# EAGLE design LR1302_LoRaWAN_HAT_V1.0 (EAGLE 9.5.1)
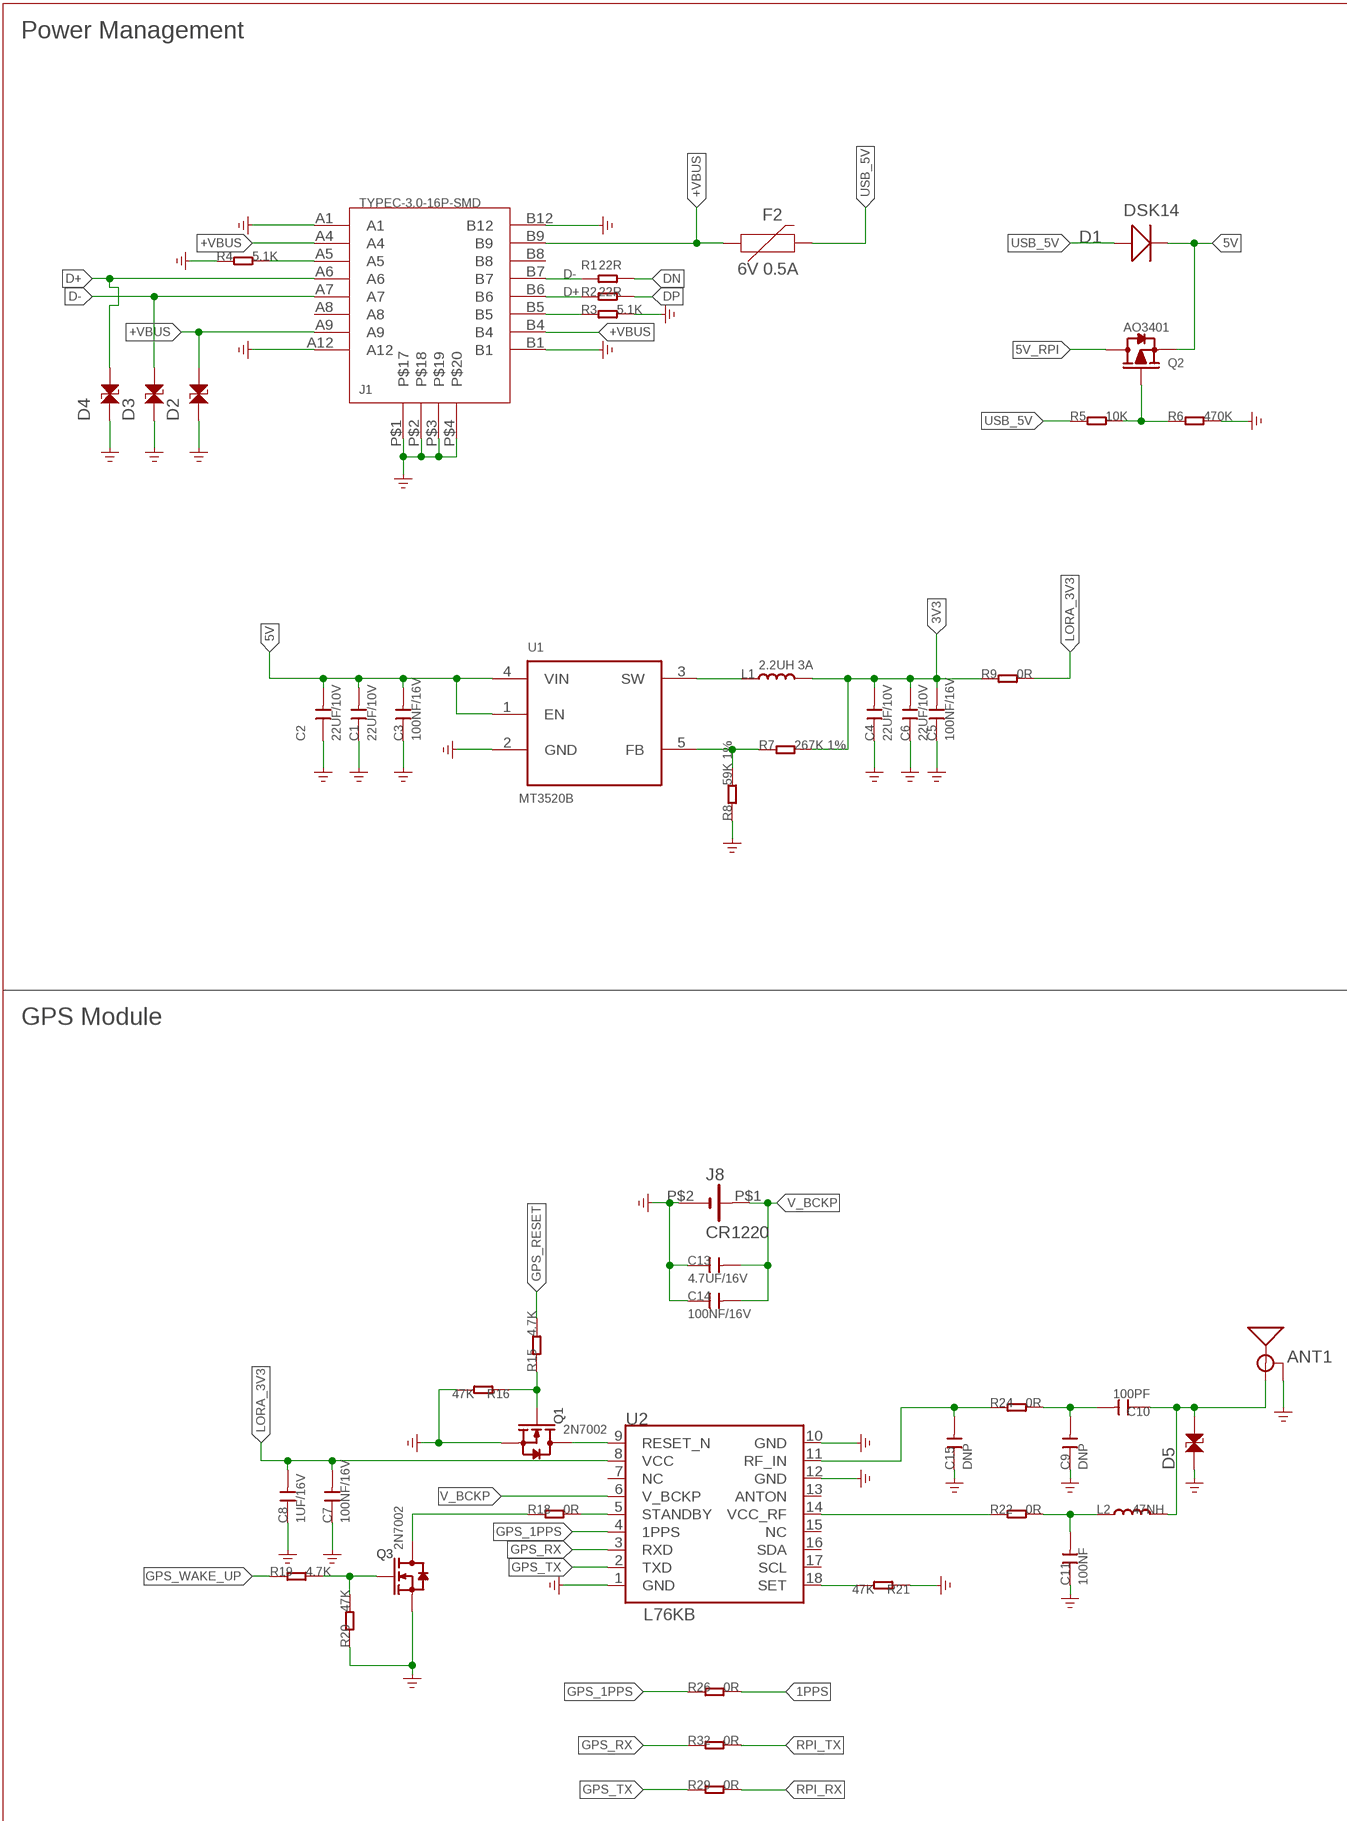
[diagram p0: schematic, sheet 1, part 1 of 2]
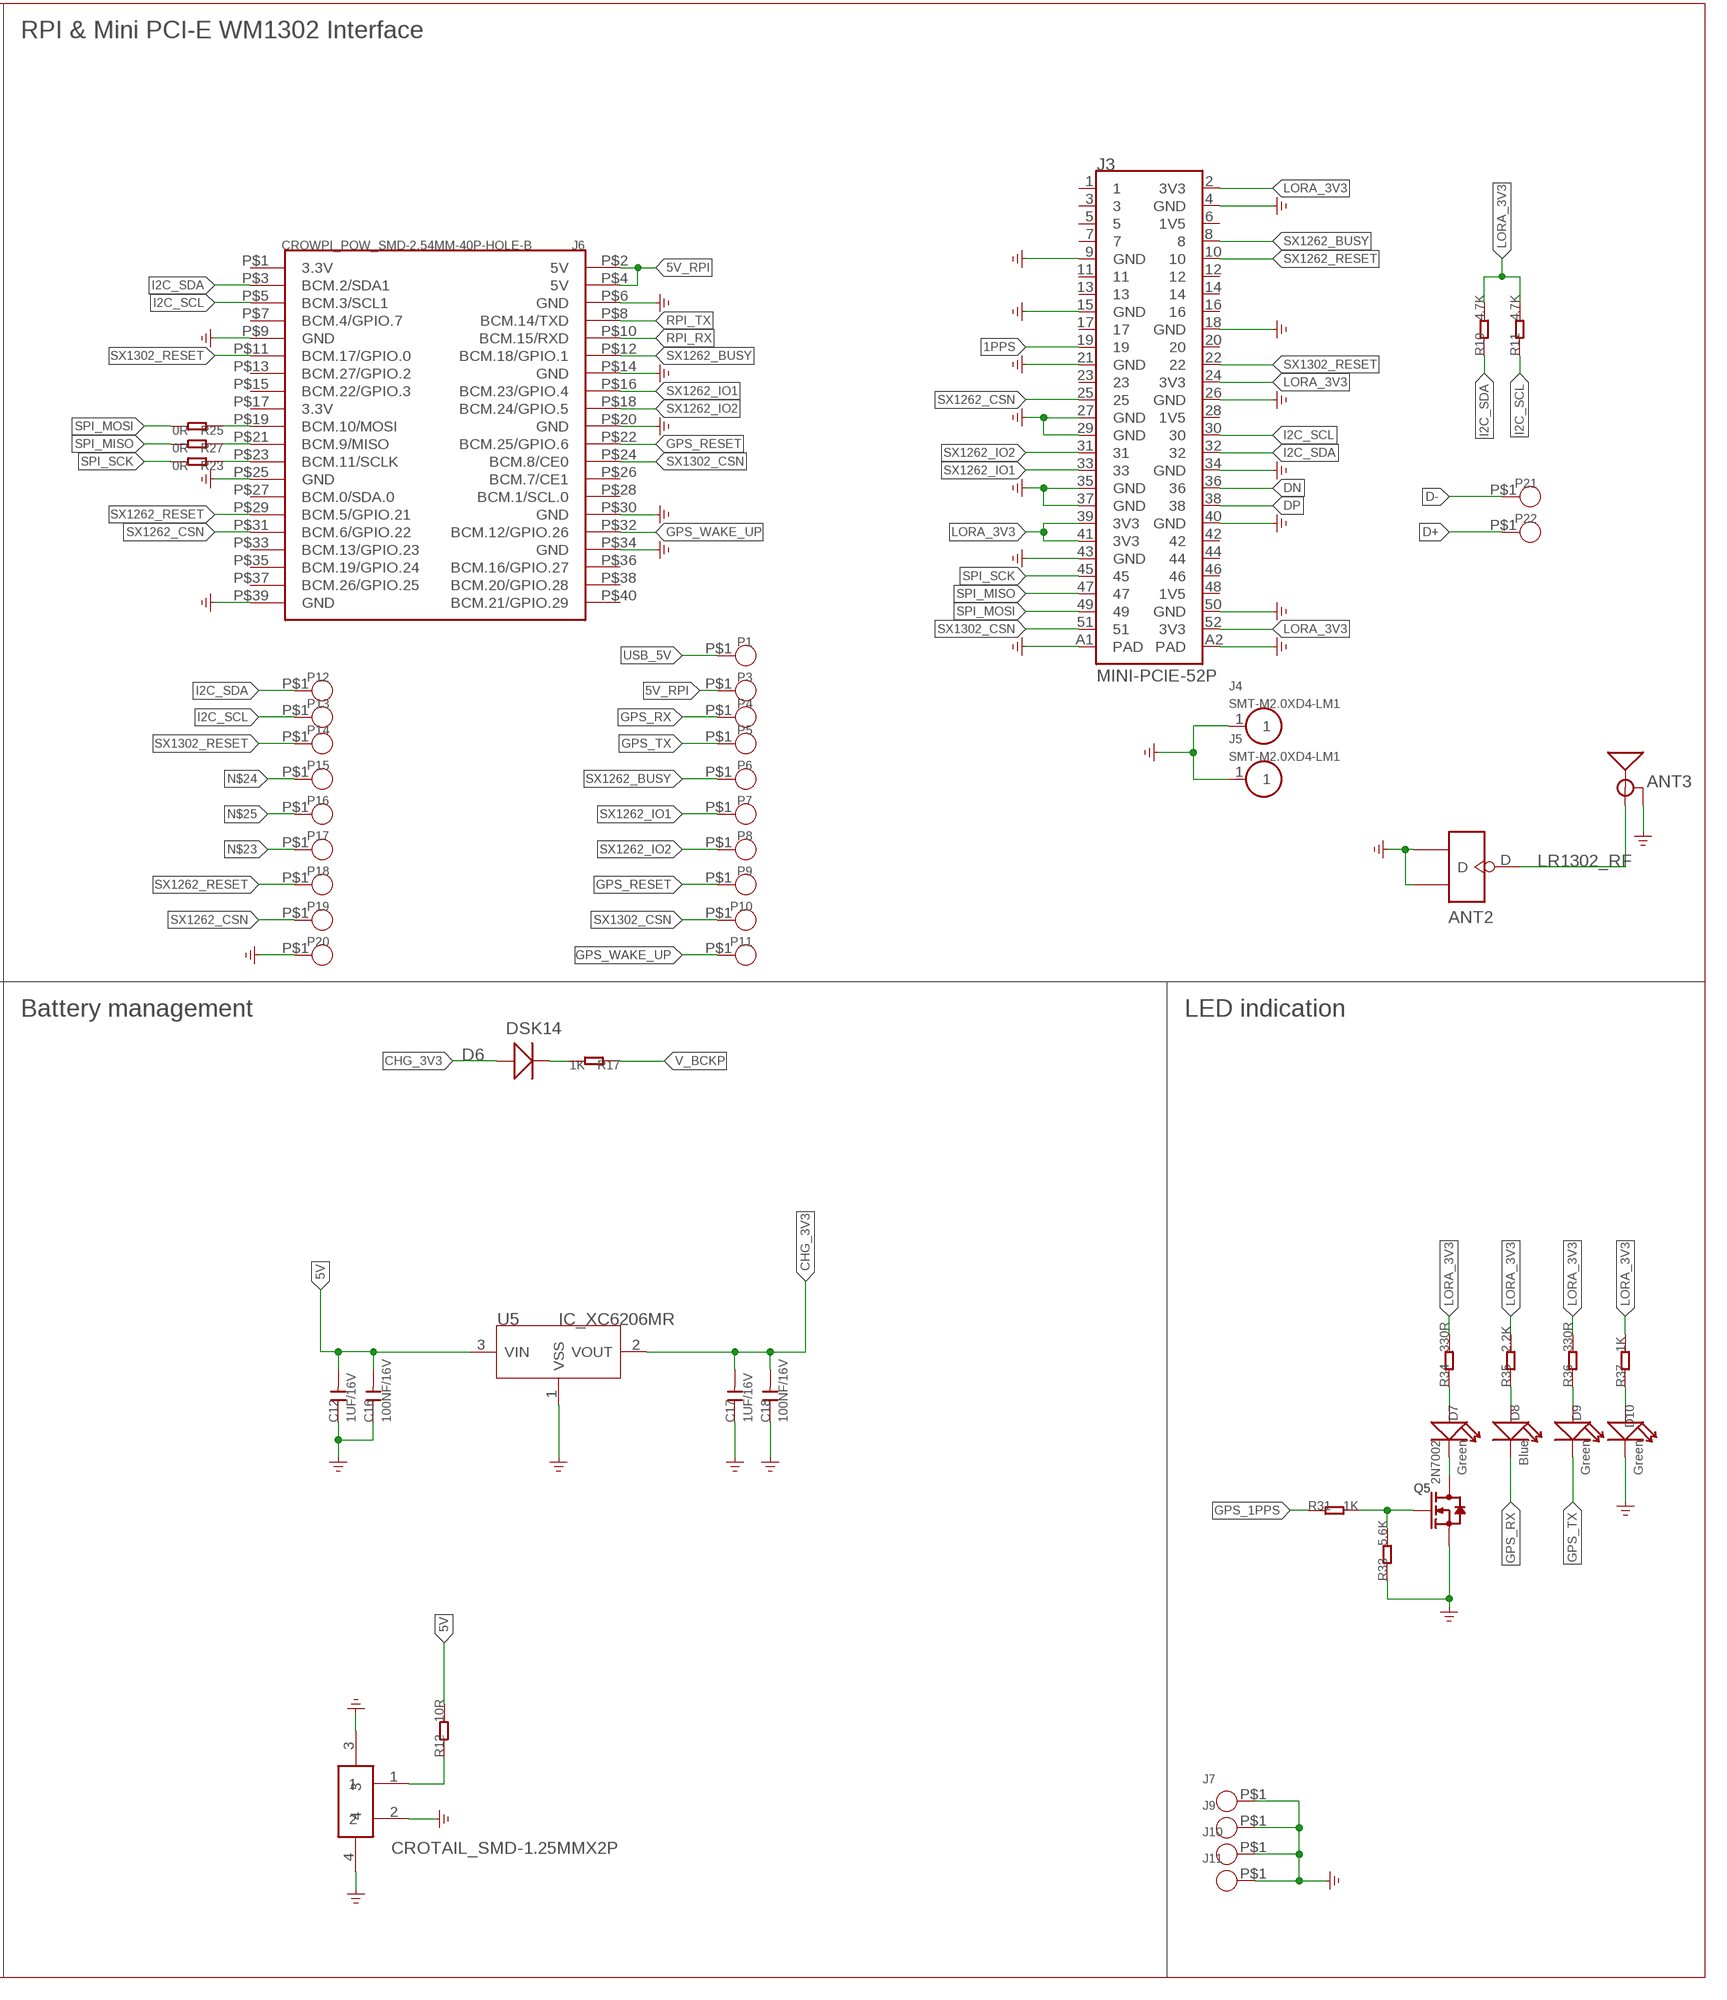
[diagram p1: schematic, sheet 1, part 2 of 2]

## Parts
ANT1  ANTENNA-SMA-GROUNDEDEDGE_SMA  [SMA-EDGE]
ANT2  CONNECTOR-NEW_ANTENNA-U-FL  [CONNECTOR-NEW_U-FL3P-SMD-2.6X2.6X1.0MM]
ANT3  ANTENNA-SMA-GROUNDEDEDGE_SMA  [SMA-EDGE]
C1  22UF/10V  C0805  [C0805]
C2  22UF/10V  C0805  [C0805]
C3  100NF/16V  C0603  [C0603]
C4  22UF/10V  C0805  [C0805]
C5  100NF/16V  C0603  [C0603]
C6  22UF/10V  C0805  [C0805]
C7  100NF/16V  C0603  [C0603]
C8  1UF/16V  C0603  [C0603]
C9  DNP  C0603  [C0603]
C10  100PF  C0603  [C0603]
C11  100NF  C0603  [C0603]
C12  1UF/16V  C0603  [C0603]
C13  4.7UF/16V  C0603  [C0603]
C14  100NF/16V  C0603  [C0603]
C15  DNP  C0603  [C0603]
C16  100NF/16V  C0603  [C0603]
C17  1UF/16V  C0603  [C0603]
C18  100NF/16V  C0603  [C0603]
D1  DSK14  DIODE  [D_SOD123FL]
D2  LXES15AAA1-153  [0402-ESD]
D3  LXES15AAA1-153  [0402-ESD]
D4  LXES15AAA1-153  [0402-ESD]
D5  LXES15AAA1-153  [0402-ESD]
D6  DSK14  DIODE  [D_SOD123FL]
D7  Green  LED-SMT0603  [LED0603]
D8  Blue  LED-SMT0603  [LED0603]
D9  Green  LED-SMT0603  [LED0603]
D10  Green  LED-SMT0603  [LED0603]
F2  6V 0.5A  PPTC_6V500MA  [0805]
J1  TYPEC-3.0-16P-SMD  [KEVIN_3.0TYPEC-SMD]
J2  CROTAIL_SMD-1.25MMX2P  [CROTAIL_SMD-1.25MMX2P]
J3  MINI-PCIE-52P  [MPCI-E0.8MM-52P-SMD]
J4  SMT-M2.0XD4-LM1  [SMD-M2.0XD4.0-LM]
J5  SMT-M2.0XD4-LM1  [SMD-M2.0XD4.0-LM]
J6  CROWPI_POW_SMD-2.54MM-40P-HOLE-B  [CROWPI_POW_SMD-2.54MM-40P-HOLE-B]
J7  PAD-HOLE  [PAD-THOD600X280]
J8  CR1220  CR1220LFCR1220-SMD  [CR1220-SMD]
J9  PAD-HOLE  [PAD-THOD600X280]
J10  PAD-HOLE  [PAD-THOD600X280]
J11  PAD-HOLE  [PAD-THOD600X280]
L1  2.2UH 3A  LL0420  [L0420]
L2  47NH  L0603  [L0603]
P1  TEST_PADPAD-1.5MM  [TEST_PAD-1.5MM]
P3  TEST_PADPAD-1.5MM  [TEST_PAD-1.5MM]
P4  TEST_PADPAD-1.5MM  [TEST_PAD-1.5MM]
P5  TEST_PADPAD-1.5MM  [TEST_PAD-1.5MM]
P6  TEST_PADPAD-1.5MM  [TEST_PAD-1.5MM]
P7  TEST_PADPAD-1.5MM  [TEST_PAD-1.5MM]
P8  TEST_PADPAD-1.5MM  [TEST_PAD-1.5MM]
P9  TEST_PADPAD-1.5MM  [TEST_PAD-1.5MM]
P10  TEST_PADPAD-1.5MM  [TEST_PAD-1.5MM]
P11  TEST_PADPAD-1.5MM  [TEST_PAD-1.5MM]
P12  TEST_PADPAD-1.5MM  [TEST_PAD-1.5MM]
P13  TEST_PADPAD-1.5MM  [TEST_PAD-1.5MM]
P14  TEST_PADPAD-1.5MM  [TEST_PAD-1.5MM]
P15  TEST_PADPAD-1.5MM  [TEST_PAD-1.5MM]
P16  TEST_PADPAD-1.5MM  [TEST_PAD-1.5MM]
P17  TEST_PADPAD-1.5MM  [TEST_PAD-1.5MM]
P18  TEST_PADPAD-1.5MM  [TEST_PAD-1.5MM]
P19  TEST_PADPAD-1.5MM  [TEST_PAD-1.5MM]
P20  TEST_PADPAD-1.5MM  [TEST_PAD-1.5MM]
P21  TEST_PADPAD-1.5MM  [TEST_PAD-1.5MM]
P22  TEST_PADPAD-1.5MM  [TEST_PAD-1.5MM]
Q1  2N7002  MOSFET-NSOT23  [MOS_SOT23]
Q2  AO3401  MOSFET-PSOT23  [PMOS_SOT23]
Q3  2N7002  MOSFET-NSOT23  [MOS_SOT23]
Q5  2N7002  MOSFET-NSOT23  [MOS_SOT23]
R1  22R  R0603  [R0603]
R2  22R  R0603  [R0603]
R3  5.1K  R0603  [R0603]
R4  5.1K  R0603  [R0603]
R5  10K  R0603  [R0603]
R6  470K  R0603  [R0603]
R7  267K 1%  R0603  [R0603]
R8  59K 1%  R0603  [R0603]
R9  0R  R0603  [R0603]
R10  4.7K  R0603  [R0603]
R11  4.7K  R0603  [R0603]
R12  10R  R0603  [R0603]
R15  4.7K  R0603  [R0603]
R16  47K  R0603  [R0603]
R17  1K  R0603  [R0603]
R18  0R  R0603  [R0603]
R19  4.7K  R0603  [R0603]
R20  47K  R0603  [R0603]
R21  47K  R0603  [R0603]
R22  0R  R0603  [R0603]
R23  0R  R0603  [R0603]
R24  0R  R0603  [R0603]
R25  0R  R0603  [R0603]
R26  0R  R0603  [R0603]
R27  0R  R0603  [R0603]
R29  0R  R0603  [R0603]
R31  1K  R0603  [R0603]
R32  0R  R0603  [R0603]
R33  5.6K  R0603  [R0603]
R34  330R  R0603  [R0603]
R35  2.2K  R0603  [R0603]
R36  330R  R0603  [R0603]
R37  1K  R0603  [R0603]
U1  MT3520B  [IC_SOT23-5]
U2  L76KB  [LCC-18]
U5  IC_XC6206MR  [IC_SOT23]

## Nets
1PPS: J3.19 R26.2
3V3: C4.2 C5.2 C6.2 L1.2 R7.2 R9.1
5V: C1.2 C2.2 C3.2 C12.2 C16.2 D1.- Q2.2(S) R12.2 U1.1(EN) U1.4(VIN) U5.3(VIN)
5V_RPI: J6.P$2(5V) J6.P$4(5V) P3.P$1 Q2.3(D)
+VBUS: D2.2 F2.1 J1.A4 J1.A9 J1.B4 J1.B9
CHG_3V3: C17.2 C18.2 D6.+ U5.2(VOUT)
D+: D4.2 J1.A6 J1.B6 P22.P$1 R2.1
D-: D3.2 J1.A7 J1.B7 P21.P$1 R1.1
DN: J3.36 R1.2
DP: J3.38 R2.2
GND: ANT1.GND@0(GND) ANT1.GND@1(GND) ANT1.GND@2(GND) ANT1.GND@3(GND) ANT2.GND1 ANT2.GND2 ANT3.GND@0(GND) ANT3.GND@1(GND) ANT3.GND@2(GND) ANT3.GND@3(GND) C1.1 C2.1 C3.1 C4.1 C5.1 C6.1 C7.1 C8.1 C9.1 C11.1 C12.1 C13.1 C14.1 C15.1 C16.1 C17.1 C18.1 D2.1 D3.1 D4.1 D5.1 D10.- J1.A1 J1.A12 J1.B1 J1.B12 J1.P$1 J1.P$2 J1.P$3 J1.P$4 J2.2 J2.3 J2.4 J3.4(GND) J3.9(GND) J3.15(GND) J3.18(GND) J3.21(GND) J3.26(GND) J3.27(GND) J3.29(GND) J3.34(GND) J3.35(GND) J3.37(GND) J3.40(GND) J3.43(GND) J3.50(GND) J3.A1(PAD) J3.A2(PAD) J4.1 J5.1 J6.P$6(GND) J6.P$9(GND) J6.P$14(GND) J6.P$20(GND) J6.P$25(GND) J6.P$30(GND) J6.P$34(GND) J6.P$39(GND) J7.P$1 J8.P$2(-) J9.P$1 J10.P$1 J11.P$1 P20.P$1 Q1.2(S) Q3.2(S) Q5.2(S) R3.2 R4.1 R6.2 R8.1 R16.2 R20.1 R21.1 R33.1 U1.2(GND) U2.1(GND) U2.10(GND) U2.12(GND) U5.1(VSS)
GPS_1PPS: R26.1 R31.1 U2.4(1PPS)
GPS_RESET: J6.P$22(BCM.25/GPIO.6) P9.P$1 R15.2
GPS_RX: D8.- P4.P$1 R32.1 U2.3(RXD)
GPS_TX: D9.- P5.P$1 R29.1 U2.2(TXD)
GPS_WAKE_UP: J6.P$32(BCM.12/GPIO.26) P11.P$1 R19.1
I2C_SCL: J3.30 J6.P$5(BCM.3/SCL1) P13.P$1 R11.1
I2C_SDA: J3.32 J6.P$3(BCM.2/SDA1) P12.P$1 R10.1
LORA_3V3: C7.2 C8.2 J3.2(3V3) J3.24(3V3) J3.39(3V3) J3.41(3V3) J3.52(3V3) R9.2 R10.2 R11.2 R34.2 R35.2 R36.2 R37.2 U2.8(VCC)
LR1302_RF: ANT2.D ANT3.SIG(SIGNAL)
N$1: J1.B5 R3.1
N$2: J1.A5 R4.2
N$3: L1.1 U1.3(SW)
N$4: R7.1 R8.2 U1.5(FB)
N$5: Q2.1(G) R5.2 R6.1
N$6: J2.1 R12.1
N$11: Q1.3(D) U2.9(RESET_N)
N$12: Q1.1(G) R15.1 R16.1
N$13: D6.- R17.2
N$14: R18.2 U2.5(STANDBY)
N$15: R21.2 U2.18(SET)
N$16: Q3.3(D) R18.1
N$17: Q3.1(G) R19.2 R20.2
N$18: C15.2 R24.1 U2.11(RF_IN)
N$19: C9.2 C10.2 R24.2
N$20: ANT1.SIG(SIGNAL) C10.1 D5.2 L2.2
N$21: R22.1 U2.14(VCC_RF)
N$22: C11.2 L2.1 R22.2
N$23: J6.P$23(BCM.11/SCLK) P17.P$1 R23.1
N$24: J6.P$19(BCM.10/MOSI) P15.P$1 R25.1
N$25: J6.P$21(BCM.9/MISO) P16.P$1 R27.1
N$27: Q5.1(G) R31.2 R33.2
N$28: D7.+ R34.1
N$29: D7.- Q5.3(D)
N$30: D8.+ R35.1
N$31: D10.+ R37.1
N$32: D9.+ R36.1
RPI_RX: J6.P$10(BCM.15/RXD) R29.2
RPI_TX: J6.P$8(BCM.14/TXD) R32.2
SPI_MISO: J3.47 R27.2
SPI_MOSI: J3.49 R25.2
SPI_SCK: J3.45 R23.2
SX1262_BUSY: J3.8 J6.P$12(BCM.18/GPIO.1) P6.P$1
SX1262_CSN: J3.25 J6.P$31(BCM.6/GPIO.22) P19.P$1
SX1262_IO1: J3.33 J6.P$16(BCM.23/GPIO.4) P7.P$1
SX1262_IO2: J3.31 J6.P$18(BCM.24/GPIO.5) P8.P$1
SX1262_RESET: J3.10 J6.P$29(BCM.5/GPIO.21) P18.P$1
SX1302_CSN: J3.51 J6.P$24(BCM.8/CE0) P10.P$1
SX1302_RESET: J3.22 J6.P$11(BCM.17/GPIO.0) P14.P$1
USB_5V: D1.+ F2.2 P1.P$1 R5.1
V_BCKP: C13.2 C14.2 J8.P$1(+) R17.1 U2.6(V_BCKP)
Unconnected: J1.A8 J1.B8 J3.1 J3.3 J3.5 J3.6(1V5) J3.7 J3.11 J3.12 J3.13 J3.14 J3.16 J3.17 J3.20 J3.23 J3.28(1V5) J3.42 J3.44 J3.46 J3.48(1V5) J6.P$1(3.3V) J6.P$7(BCM.4/GPIO.7) J6.P$13(BCM.27/GPIO.2) J6.P$15(BCM.22/GPIO.3) J6.P$17(3.3V) J6.P$26(BCM.7/CE1) J6.P$27(BCM.0/SDA.0) J6.P$28(BCM.1/SCL.0) J6.P$33(BCM.13/GPIO.23) J6.P$35(BCM.19/GPIO.24) J6.P$36(BCM.16/GPIO.27) J6.P$37(BCM.26/GPIO.25) J6.P$38(BCM.20/GPIO.28) J6.P$40(BCM.21/GPIO.29) U2.7(NC) U2.13(ANTON) U2.15(NC) U2.16(SDA) U2.17(SCL)

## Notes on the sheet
- Power Management | RPI & Mini PCI-E WM1302 Interface
- GPS Module | Battery management | LED indication

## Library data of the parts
ANT1 ANT3 = WM1302_Raspberry_Pi _Hat:ANTENNA-SMA-GROUNDED: SMA Antenna Connector w/ Ground; PROD_ID: CONN-08289
ANT2 = WM1302_Raspberry_Pi _Hat:CONNECTOR-NEW_ANTENNA-U-FL: 320110048
C1 C2 C4 C6 = WM1302_Raspberry_Pi _Hat:C0805
C3 C5 C7-C18 = WM1302_Raspberry_Pi _Hat:C0603
D1 D6 = WM1302_Raspberry_Pi _Hat:DIODE*
D2-D5 = WM1302_Raspberry_Pi _Hat:LXES15AAA1-153
D7-D10 = WM1302_Raspberry_Pi _Hat:LED-SMT*
F2 = WM1302_Raspberry_Pi _Hat:PPTC: Resettable Fuse PPTC; PROD_ID: RES-13945
J1 = WM1302_Raspberry_Pi _Hat:TYPEC-3.0-16P-SMD
J2 = WM1302_Raspberry_Pi _Hat:CROTAIL_SMD-1.25MMX2P
J3 = WM1302_Raspberry_Pi _Hat:MINI-PCIE-52P
J4 J5 = WM1302_Raspberry_Pi _Hat:SMT-M2.0XD4-LM1
J6 = WM1302_Raspberry_Pi _Hat:CROWPI_POW_SMD-2.54MM-40P-HOLE-B
J7 J9-J11 = WM1302_Raspberry_Pi _Hat:PAD-HOLE
J8 = WM1302_Raspberry_Pi _Hat:CR1220LF: Battery Holder, SMT, 12mm
L1 L2 = WM1302_Raspberry_Pi _Hat:L*
P1 P3-P22 = WM1302_Raspberry_Pi _Hat:TEST_PAD*
Q1 Q3 Q5 = WM1302_Raspberry_Pi _Hat:MOSFET-N*: IRLL014: http://www.vishay.com/docs/91319/sihll014.pdf
Q2 = WM1302_Raspberry_Pi _Hat:MOSFET-P: IRLL014: http://www.vishay.com/docs/91319/sihll014.pdf
R1-R12 R15-R27 R29 R31-R37 = WM1302_Raspberry_Pi _Hat:R0603
U1 = WM1302_Raspberry_Pi _Hat:MT3520B
U2 = WM1302_Raspberry_Pi _Hat:L76KB
U5 = WM1302_Raspberry_Pi _Hat:IC_XC6206: LOW ESR Cap.Compatible Positive Voltage Regulators

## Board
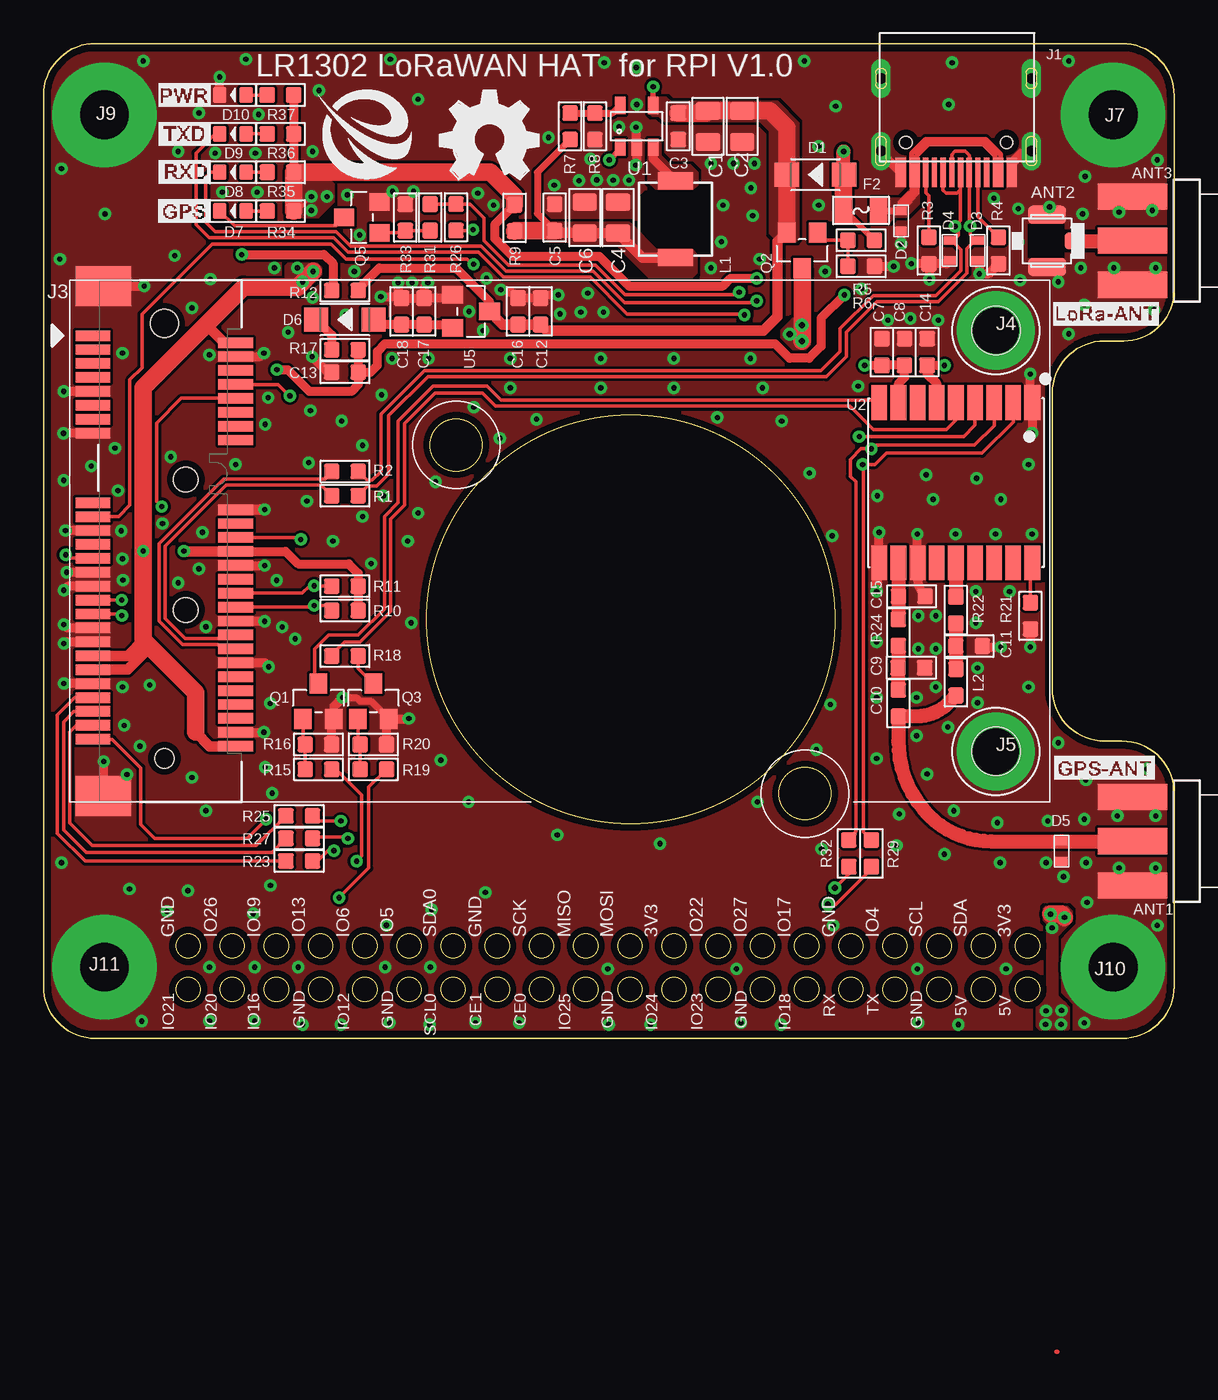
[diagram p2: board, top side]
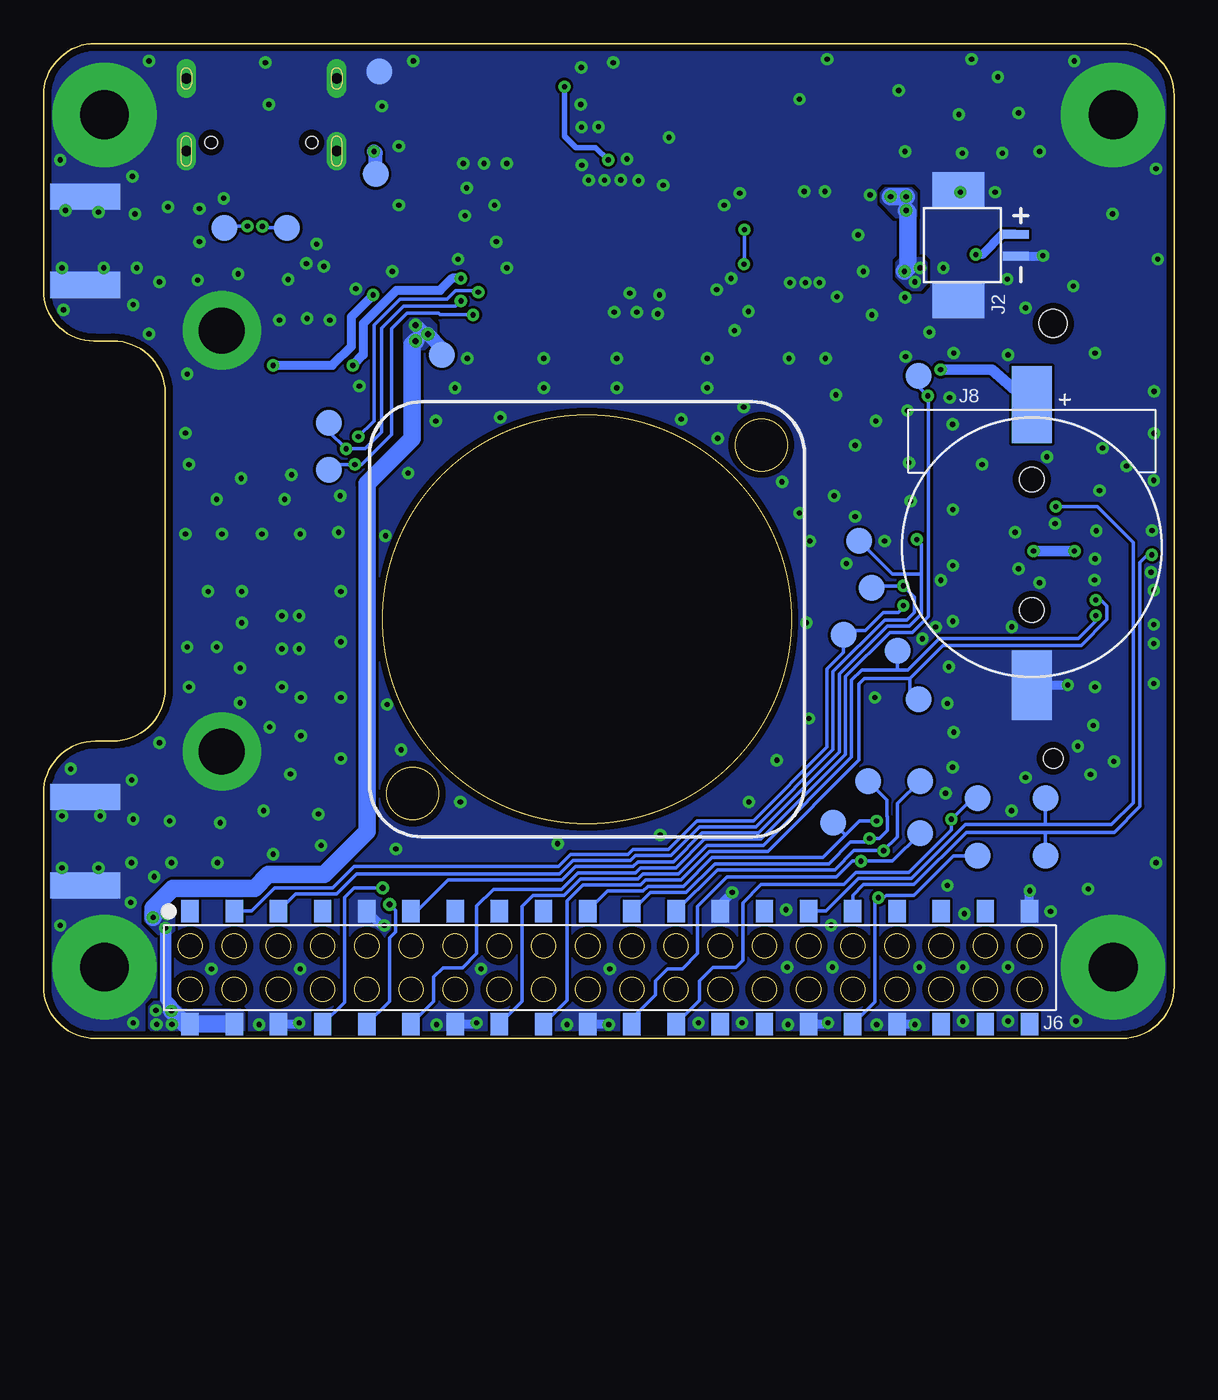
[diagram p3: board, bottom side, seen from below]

Size 65 x 57.2 mm. Coordinates in mm from the lower left corner, seen from the top.
Outline: 0,3 0,54.2 arc-90 3,57.2 62,57.2 arc-90 65,54.2 65,43 arc-90 62.1,40.1 61,40.1 arc90 58,37.1 58,20.1 arc90 61,17.1 62,17.1 arc-90 65,14.1 65,3 arc-90 62,0 3,0 arc-90 0,3
Outline: circle at 33.75,24.1 radius 11.75
Outline: circle at 23.73,34.12 radius 1.5
Outline: circle at 43.78,14.08 radius 1.5
Copper layers (1*16): Top 0.035mm / dielectric 1.5mm / Bottom 0.035mm
Design rules "default *": minimum track width 5mil, minimum drill 0.3mm, track to track 6mil, track to pad 6mil, pad to pad 6mil, via to via 6mil, smd to smd 6mil, copper to edge 15mil, drill to drill 6mil, minimum pad ring 10mil, minimum via ring 8mil, stop-mask expansion 4mil, vias tented up to drill 100mil, thermal gap 10mil
tRestrict: 19 lines

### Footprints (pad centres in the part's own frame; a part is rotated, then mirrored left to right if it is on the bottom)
SMA-EDGE = smd 1.5 x 4: GND@0 -2.54,0; GND@1 2.54,0; SIG 0,0 | smd 1.5 x 4 bottom: GND@2 -2.54,0; GND@3 2.54,0
CONNECTOR-NEW_U-FL3P-SMD-2.6X2.6X1.0MM = smd 1.05 x 1: D -1.524,0 | smd 2.2 x 1.05: GND1 0,1.5; GND2 0,-1.5
C0805 = smd 1.016 x 1.397: 1 -0.889,0; 2 0.889,0
C0603 = smd 0.889 x 0.889: 1 -0.762,0; 2 0.762,0
D_SOD123FL = smd 1.397 x 1.397: + -1.651,0; - 1.651,0
0402-ESD = smd 0.5 x 0.7: 1 -0.58,0; 2 0.58,0
LED0603 = smd 0.762 x 0.889: + -0.762,0; - 0.762,0
0805 = smd 1 x 1.4: 1 -1,0; 2 1,0
KEVIN_3.0TYPEC-SMD = smd 0.3 x 1.7: A1 -3.35,0.5; A4 -2.55,0.5; A5 -1.25,0.5; A6 -0.25,0.5; A7 0.25,0.5; A8 1.25,0.5; A9 2.55,0.5; A12 3.35,0.5; B1 3.05,0.5; B4 2.25,0.5; B5 1.75,0.5; B6 0.75,0.5; B7 -0.75,0.5; B8 -1.75,0.5; B9 -2.25,0.5; B12 -3.05,0.5 | drill 0.6 pad 1.016 long: P$1 -4.325,-0.72; P$2 4.325,-0.72; P$3 -4.325,-4.9; P$4 4.325,-4.9 | hole 0.68: -2.89,-1.22; 2.89,-1.22
CROTAIL_SMD-1.25MMX2P = smd 0.5 x 1.5: 1 -0.625,2; 2 0.625,2 | smd 2 x 3: 3 -3.2,-1.3; 4 3.2,-1.3
MPCI-E0.8MM-52P-SMD = smd 0.6 x 2: 1 -11.8,-4.1; 2 -11.4,4.1; 3 -11,-4.1; 4 -10.6,4.1; 5 -10.2,-4.1; 6 -9.8,4.1; 7 -9.4,-4.1; 8 -9,4.1; 9 -8.6,-4.1; 10 -8.2,4.1; 11 -7.8,-4.1; 12 -7.4,4.1; 13 -7,-4.1; 14 -6.6,4.1; 15 -6.2,-4.1; 16 -5.8,4.1; 17 -2.2,-4.1; 18 -1.8,4.1; 19 -1.4,-4.1; 20 -1,4.1; 21 -0.6,-4.1; 22 -0.2,4.1; 23 0.2,-4.1; 24 0.6,4.1; 25 1,-4.1; 26 1.4,4.1; 27 1.8,-4.1; 28 2.2,4.1; 29 2.6,-4.1; 30 3,4.1; 31 3.4,-4.1; 32 3.8,4.1; 33 4.2,-4.1; 34 4.6,4.1; 35 5,-4.1; 36 5.4,4.1; 37 5.8,-4.1; 38 6.2,4.1; 39 6.6,-4.1; 40 7,4.1; 41 7.4,-4.1; 42 7.8,4.1; 43 8.2,-4.1; 44 8.6,4.1; 45 9,-4.1; 46 9.4,4.1; 47 9.8,-4.1; 48 10.2,4.1; 49 10.6,-4.1; 50 11,4.1; 51 11.4,-4.1; 52 11.8,4.1 | smd 2.3 x 3.2: A1 -14.65,-3.5; A2 14.65,-3.5 | hole 1.1: 12.5,0 | hole 1.6: -12.5,0
SMD-M2.0XD4.0-LM = drill 2.65 pad 4.5: 1 0,0
CROWPI_POW_SMD-2.54MM-40P-HOLE-B = smd 1 x 1.3 bottom: P$1 -24.073,-3.227; P$2 -24.073,3.273; P$3 -21.533,-3.227; P$4 -21.533,3.273; P$5 -18.993,-3.227; P$6 -18.993,3.273; P$7 -16.453,-3.227; P$8 -16.453,3.273; P$9 -13.913,-3.227; P$10 -13.913,3.273; P$11 -11.373,-3.227; P$12 -11.373,3.273; P$13 -8.833,-3.227; P$14 -8.833,3.273; P$15 -6.293,-3.227; P$16 -6.293,3.273; P$17 -3.753,-3.227; P$18 -3.753,3.273; P$19 -1.213,-3.227; P$20 -1.213,3.273; P$21 1.327,-3.227; P$22 1.327,3.273; P$23 3.867,-3.227; P$24 3.867,3.273; P$25 6.407,-3.227; P$26 6.407,3.273; P$27 8.947,-3.227; P$28 8.947,3.273; P$29 11.487,-3.227; P$30 11.487,3.273; P$31 14.027,-3.227; P$32 14.027,3.273; P$33 16.567,-3.227; P$34 16.567,3.273; P$35 19.107,-3.227; P$36 19.107,3.273; P$37 21.647,-3.227; P$38 21.647,3.273; P$39 24.187,-3.227; P$40 24.187,3.273
PAD-THOD600X280 = drill 2.8 pad 6: P$1 0,0
CR1220-SMD = smd 2.3 x 4.4: P$1 0,8.2 | smd 2.3 x 4: P$2 0,-7.925 | hole 1.4: 0,3.9; 0,-3.6
L0420 = smd 2 x 1: 1 0,2.2; 2 0,-2.2
L0603 = smd 0.889 x 0.889: 1 -0.762,0; 2 0.762,0
TEST_PAD-1.5MM = smd 1.5 x 1.5: P$1 0,0
MOS_SOT23 = smd 1.016 x 1.143: 1 -0.889,-1.016; 2 0.889,-1.016; 3 0,1.016
PMOS_SOT23 = smd 1.016 x 1.143: 1 -0.889,-1.016; 2 0.889,-1.016; 3 0,1.016
R0603 = smd 0.889 x 0.889: 1 -0.762,0; 2 0.762,0
IC_SOT23-5 = smd 0.6 x 1: 1 -0.95,-1.2; 2 0,-1.2; 3 0.95,-1.2; 4 0.95,1.2; 5 -0.95,1.2
LCC-18 = smd 2 x 0.9: 1 -4.6,4.4; 2 -4.6,3.3; 3 -4.6,2.2; 4 -4.6,1.1; 5 -4.6,0; 6 -4.6,-1.1; 7 -4.6,-2.2; 8 -4.6,-3.3; 9 -4.6,-4.4; 10 4.6,-4.4; 11 4.6,-3.3; 12 4.6,-2.2; 13 4.6,-1.1; 14 4.6,0; 15 4.6,1.1; 16 4.6,2.2; 17 4.6,3.3; 18 4.6,4.4
IC_SOT23 = smd 1.016 x 1.2: 1 -0.95,-1.06; 2 0.95,-1.06; 3 0,1.06

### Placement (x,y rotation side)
ANT1  62.6,11.34 270 top
ANT2  57.69,45.85 180 top
ANT3  62.6,45.86 270 top
C1  38.2,52.44 90 top
C2  40.17,52.44 90 top
C3  36.49,52.44 90 top
C4  33.04,47.19 270 top
C5  29.39,47.19 270 top
C6  31.12,47.19 270 top
C7  48.2,39.46 270 top
C8  49.5,39.46 270 top
C9  49.89,21.31 180 top
C10  49.14,19.28 90 top
C11  53.21,22.56 180 top
C12  28.58,41.8 270 top
C13  17.33,38.3 0 top
C14  50.8,39.46 270 top
C15  49.92,25.42 180 top
C16  27.28,41.8 270 top
C17  21.88,41.8 270 top
C18  20.58,41.8 270 top
D1  44.38,49.66 180 top
D2  49.3,47 90 top
D3  53.7,45.3 90 top
D4  52.1,45.3 90 top
D5  58.52,10.76 90 top
D6  17.33,41.33 180 top
D7  10.9,47.57 180 top
D8  10.9,49.8 180 top
D9  10.9,52 180 top
D10  10.89,54.24 180 top
F2  47,47.6 180 top
J1  52.47,50.29 180 top
J2  11.1,45.6 270 bottom
J3  6.95,28.6 270 top
J4  54.75,40.7 0 top
J5  54.75,16.5 0 top
J6  32.5,4.1 180 top
J7  61.5,53.1 0 top
J8  8.18,28.24 0 bottom
J9  3.5,53.1 0 top
J10  61.5,4.1 0 top
J11  3.5,4.1 0 top
L1  36.33,47.09 0 top
L2  52.46,20.48 270 top
P1  45.9,49.7 0 bottom
P3  42.1,39.3 270 bottom
P4  48.6,35.4 270 bottom
P5  48.6,32.7 270 bottom
P6  14.7,38.1 270 bottom
P7  15.9,22.3 270 bottom
P8  14.7,19.5 270 bottom
P9  14.6,11.8 270 bottom
P10  11.3,13.8 270 bottom
P11  11.3,10.5 270 bottom
P12  19,23.2 270 bottom
P13  17.4,25.9 270 bottom
P14  18.1,28.6 270 bottom
P15  19.6,12.4 270 bottom
P16  17.6,14.8 270 bottom
P17  14.6,14.8 270 bottom
P18  7.4,13.8 270 bottom
P19  7.4,10.5 270 bottom
P20  45.7,55.6 270 bottom
P21  54.6,46.6 270 bottom
P22  51,46.6 270 bottom
Q1  15.81,19.39 0 top
Q2  43.62,45.31 180 top
Q3  18.96,19.39 0 top
Q5  18.31,47.2 90 top
R1  17.33,31.2 180 top
R2  17.33,32.6 180 top
R3  50.9,45.3 270 top
R4  54.9,45.3 90 top
R5  47.01,45.89 180 top
R6  47.01,44.39 0 top
R7  30.28,52.44 270 top
R8  31.7,52.44 90 top
R9  27.09,47.17 90 top
R10  17.33,24.6 0 top
R11  17.33,26 0 top
R12  17.33,43 0 top
R15  15.81,15.47 0 top
R16  15.81,16.9 0 top
R17  17.33,39.59 180 top
R18  17.33,21.99 180 top
R19  18.96,15.47 180 top
R20  18.96,16.9 180 top
R21  56.74,24.29 90 top
R22  52.45,24.63 270 top
R23  14.7,10.2 180 top
R24  49.14,23.34 270 top
R25  14.7,12.8 180 top
R26  23.71,47.21 270 top
R27  14.7,11.5 180 top
R29  47.6,10.64 270 top
R31  22.23,47.2 270 top
R32  46.3,10.64 270 top
R33  20.8,47.2 270 top
R34  13.63,47.57 0 top
R35  13.63,49.8 0 top
R36  13.63,52 0 top
R37  13.62,54.24 0 top
U1  34.1,52.44 0 top
U2  52.45,31.95 270 top
U5  24.58,41.8 270 top
U$49  [OSHW_FILLX200_NOTEXT]  22.8,49.4 0 top
U$50  [ELECROW-NEW]  15.74,49.4 0 top

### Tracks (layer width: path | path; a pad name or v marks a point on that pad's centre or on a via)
1PPS  (via drill 0.3 pad 0.6)
  Top 0.2: J3.19 4.31,30 4.97,30.66 4.97,37.87 5.67,38.57 5.67,41.63 9.71,45.67 16.53,45.67 17.4,44.8 24.34,44.8 24.63,44.52 v24.73,44.52 | R26.2 24.65,46.45 v24.7,46.5
  Bottom 0.2: v24.7,46.5 24.7,44.54 v24.73,44.52
3.3V
  Top 0.254: 58.23,-18 58.28,-18
3V3
  Top 0.406: R7.2 28.4,49.8 28.4,47.42 C5.2
  Top 0.61: L1.2 34.45,44.89 C4.2 C6.2 29.51,46.31 C5.2
  Top 1.016: R9.1 27.11,46.43 C5.2
  pour Top (no thermals): 37.26,45.38 35.22,45.38 33.83,46.77 33.67,46.93 29.28,46.93 29.21,46.93 28.96,46.68 28.96,45.95 29.05,45.86 29.13,45.78 29.91,45.78 30.15,45.78 30.36,45.57 32.99,45.57 33.89,44.67 34.82,43.74 37.28,43.74 37.58,44.04 37.58,44.74 37.58,45.07 37.27,45.38
5V  (via drill 0.3 pad 0.6)
  Top 0.305: U1.1 33.15,51.12 v32.53,50.5 | v35.05,54.72 U1.4
  Top 0.508: 18.16,43.16 R12.2 18.09,43.09 19.3,44.29 23.71,44.29 25.64,42.36 U5.3
  Top 0.61: Q2.2 42.2,45.8 42.2,41.5 41.4,40.7 28.92,40.7 C12.2 C16.2 26.4,41.04 U5.3
  Top 1.016: C3.2 38.07,53.2 C1.2 C2.2 41.78,53.32 42.73,52.37 D1.- Q2.2
  Bottom 0.305: v32.53,50.5 33.25,51.22 34.39,51.22 35.05,51.88 v35.05,54.72
  pour Top (no thermals): 42.25,45.78 41.73,46.3 41.73,48.31 41.73,52.19 41.22,52.7 35.72,52.7 35.39,53.03 34.99,53.03 34.98,53.04 34.78,53.24 34.78,53.31 34.78,53.94 34.95,54.11 35.79,54.11 36.02,53.88 42.19,53.88 43.44,52.63 43.44,46 43.23,45.79 43.22,45.78
5V_RPI  (via drill 0.3 pad 0.6, 0.35)
  Top 1.016: Q2.3 43.62,40.12 v43.6,40.1 | v57.9,7.15 58.51,7.15 v58.7,6.96
  Bottom 0.65: v57.64,1.59 57.64,1.9 57.98,2.24 57.98,6.28 57.99,6.29 v57.99,6.35 v57.98,6.36
  Bottom 0.813: v43.6,41 43.1,40.5 v42.9,40.5 42.1,39.7 P3.P$1
  Bottom 1.016: J6.P$4 J6.P$2 56.88,0.83 v57.64,1.59 | v43.6,40.1 43.8,39.9 43.8,34.5 46.4,31.9 46.4,11.9 48.88,9.42 52.08,9.42 52.86,8.64 57.56,8.64 58.7,7.5 v58.7,6.96
  other vias: 58.53,1.62 58.5,0.81 57.61,0.81
  pour Bottom (no thermals): 53.68,1.69 57.04,1.69 57.35,2 57.47,2.12 58.37,2.12 58.65,2.12 58.96,1.81 58.96,0.61 58.71,0.36 58.57,0.22 55.85,0.22 53.61,0.22 53.43,0.4 53.43,1.44
  pour Top (no thermals): 57.09,0.84 57.09,1.82 57.34,2.07 57.39,2.12 58.65,2.12 58.98,1.79 58.98,0.58 58.68,0.28 57.52,0.28 57.09,0.71 57.09,0.82
  pour Top (no thermals): 57.67,6.62 57.67,2.42 57.19,1.94 57.1,1.85 57.1,0.66 57.47,0.29 57.67,0.29 58.7,0.29 58.93,0.52 58.98,0.57 58.98,1.73 58.98,1.78 58.65,2.11 58.31,2.45 58.31,2.49 58.31,5.91 58.67,6.27 59.16,6.76 59.16,6.96 59.16,7.29 59.02,7.43 58.85,7.6 57.69,7.6 57.63,7.6 57.47,7.44 57.47,6.82
  pour Bottom (no thermals): 57.68,6 57.46,6.22 57.46,7.34 57.46,7.43 57.64,7.61 58.86,7.61 58.87,7.6 59.17,7.3 59.17,6.85 59.17,6.75 59.11,6.69 58.4,5.98 57.71,5.98
  pour Bottom (no thermals): 42.4,41 42.4,40.3 43.1,39.6 43.9,39.6 44.3,40 44.3,41 43.9,41.4 42.8,41.4
  pour Top (no thermals): 42.4,40.3 42.4,40.7 42.9,41.2 43.1,41.4 43.7,41.4 43.8,41.4 44.1,41.1 44.1,39.9 43.8,39.6 43.3,39.6 43.1,39.6
+VBUS
  Top 0.3: 49.74,48.5 49.92,48.68 J1.A9 49.92,50.89 50.72,51.69 54.16,51.69 55.02,50.83 J1.A4 | 49.8,48.2 50.22,48.62 J1.B4 50.22,50.79 50.83,51.4 54.06,51.4 54.72,50.74 J1.B9
  Top 0.406: 49.8,48.2 49.3,47.7 | 49.3,47.7 D2.2 48.02,47.58 F2.1 | 49.74,48.5 49.3,48.06 49.3,47.7
  pour Top (no thermals): 49.78,48.78 49.31,48.31 47.9,48.31 47.73,48.31 47.53,48.11 47.53,47.06 47.7,46.89 48.59,46.89 48.91,47.21 49.57,47.21 50.02,47.66 50.36,48 50.36,48.54 50.1,48.8 49.8,48.8
CHG_3V3
  Top 0.508: U5.2 23.35,41.02 21.9,41.02 | C17.2 C18.2 19.27,41.04 D6.+
  Top 0.61: 21.9,41.02 C17.2
D+  (via drill 0.3 pad 0.6)
  Top 0.2: R2.1 18.59,32.1 18.9,32.1 19.4,32.6 19.4,35.9 21.9,38.4 44.7,38.4 45.8,39.5 45.8,40.8 47.7,42.7 51.3,42.7 52.73,44.13 52.73,45.35 52.25,45.83 52.61,46.19 52.61,46.29 | J1.A6 52.72,48.8 | 52.61,46.29 52.61,46.49 v52.41,46.69 52.72,47 52.72,48.8 | J1.B6 51.72,48.78 51.9,48.6 52.52,48.6 52.72,48.8 | 52.61,46.29 52.2,45.88 D4.2
  Bottom 0.2: v52.41,46.69 52.32,46.6 P22.P$1
D-  (via drill 0.3 pad 0.6)
  Top 0.2: R1.1 18.64,31.75 19.15,31.75 19.85,32.45 19.85,35.8 22.1,38.05 45,38.05 46.15,39.2 46.15,40.6 47.9,42.35 51.45,42.35 53.1,44 53.1,45.4 53.58,45.88 D3.2 53.6,45.88 53.28,46.2 v53.28,46.7 53.22,46.76 J1.B7 53.22,50.78 53,51 52.4,51 52.22,50.82 J1.A7
  Bottom 0.2: v53.28,46.7 54.5,46.7 P21.P$1
DN
  Top 0.2: J3.36 10.25,23.2 10.05,23 8.15,23 7,24.15 7,25.13 7,28.3 10.5,31.8 15.97,31.8 R1.2
DP
  Top 0.2: J3.38 10.25,22.4 10,22.65 8,22.65 6.65,24.01 6.65,28.45 10.35,32.15 16.2,32.15 16.57,32.52 R2.2
GND  (via drill 0.3 pad 0.6)
  Top 0.3: J1.A12 48.15,50.77 J1.P$2 48.2,51.01 J1.B1 | J1.A1 55.82,50.29 56.55,51.01 J1.P$1 56.18,51.01 55.52,50.35 J1.B12
  Top 0.406: v17.2,19.6 18,19.6 18.2,19.4 18.82,19.4 Q3.2
  Top 0.508: v34.05,50.21 34.1,50.26 U1.2 34.07,51.27 v34.07,52.39 | J3.9 v1.16,37.2 | J3.15 v1.16,34.8 v1.15,34.79 | J3.21 v1.27,29.2 | J3.27 v1.33,26.8 | J3.29 1.4,26 v1.17,25.77 | J3.35 1.37,23.6 v1.17,23.8 | J3.37 1.27,22.8 v1.17,22.7 | J3.43 v1.18,20.4 v1.17,20.41 | J3.A2 v3.45,15.92 v3.46,15.93 | J3.50 v12.67,17.6 | J3.40 12.72,21.6 v12.95,21.37 | J3.34 12.7,24 v12.72,23.98 | J3.26 v12.71,27.2 v12.72,27.19 | R6.2 v48.87,44.39 v48.88,44.38 | D2.1 v49.3,45.67 | R3.2 49.9,44.54 v49.89,44.55 | D3.1 53.81,44.61 v53.81,43.95 54.31,43.95 R4.1 | R3.2 50.93,44.51 v50.93,43.64 | D4.1 51.92,44.54 R3.2 | J3.4 12.47,39.2 v12.67,39.4 | J3.A1 v5.79,43.25 | D10.- v10.13,55.27 | 20.67,48.09 R33.1 | R16.2 16.57,18.25 Q1.2 16.7,19.1 v17.2,19.6 | R20.1 19.73,18.25 Q3.2 20.97,18.37 v21,18.4 | v50.24,29 50.24,27.37 arc45 U2.12 50.25,26.46 arc45 C15.1 | U2.10 arc-45 48.04,27.37 v48.04,29.1 | R21.1 v56.74,22.5 | C11.1 arc45 54.12,22.5 v55.04,22.5 | v56.74,38.2 56.74,36.82 arc45 U2.1 56.85,34.82 arc-45 v56.84,34.8 | C18.1 arc-45 20.39,43.02 v20.39,43.45 | C17.1 21.88,42.94 arc-45 v22.09,43.45 | U5.1 arc-45 23.07,42.56 C17.1 | C18.1 C17.1 | v26.29,43.05 arc-45 27.15,42.7 C16.1 C12.1 arc-45 29.03,42.75 v29.59,42.75 | v19.39,42.65 20.37,42.65 arc-45 C18.1 | C13.1 16.34,38.3 v15.44,39.2
  Top 0.61: J3.18 v12.71,30.4 v12.72,30.41 | U2.10 47.9,27.2 v47.9,25.7
  Bottom 0.508: J8.P$2 v6.12,20.32 v6.11,20.32 | J6.P$39 8.31,8.49 v8.3,8.5 | J6.P$34 14.93,0.83 v14.9,0.8 | J6.P$30 19.97,0.83 v19.9,0.9 | J6.P$25 26.09,7.71 v25.4,8.4 | J6.P$20 32.53,0.83 v32.5,0.8 | J6.P$14 40.17,0.83 v40.1,0.9 | J6.P$9 45.59,6.5 v45.4,6.5 | J6.P$6 50.37,0.83 v50.3,0.9 | J2.2 7.57,44.98 v7.54,45
  other vias: 31.45,50.56 29.37,49.06 30.79,49.32 31.81,49.35 32.75,49.34 33.66,49.34 42.4,0.8 52.6,0.8 34.9,0.8 22.2,0.8 17.1,0.8 7.1,7.3 52.34,13.1 57.74,12.5 59.84,12.6 57.64,10.1 59.94,10.1 56.64,20.2 20.94,28.6 16.64,28.6 15.14,30.9 9.14,29.1 8.94,27 15.24,33.1 15.34,36.1 11.04,33 12.74,35.3 6.84,29.6 7.74,26.2 48.54,41.3 44.94,44.1 51.44,41.3 59.74,47.4 54.64,48.3 56.14,43.6 56.84,29 58.94,40.5 63.94,44.3 61.54,44.3 59.64,44.3 58.34,43.5 56.04,45.8 56.04,47.7 57.84,47.8 61.84,47.5 63.74,47.6 64.04,50.5 58.94,56.2 52.24,56.1 43.74,56.2 32.24,56.1 19.94,56.3 11.64,56.3 5.74,56.2 29.04,51.8 15.84,54.5 7.74,51 8.94,53.2 1.04,50 0.94,44.8 8.54,42 4.54,39.4 9.54,39.3 4.64,18 5.54,16.8 4.54,20.2 8.54,15 9.34,13.1 12.74,15.6 13.14,14.1 1.04,10.1 13.04,8.8 4.94,8.6 5.64,1 9.54,1 12.14,1 24.84,0.9 27.34,0.9 22.24,4.1 19.64,4.1 14.64,4.1 9.54,4.1 12.14,4.1 32.44,4 39.84,4 50.24,4 55.34,4 58.64,9.3 59.84,0.9 64.04,6.5 61.84,9.8 63.94,9.8 61.74,12.8 63.94,12.8 63.44,15.5 58.34,17 21.54,54 45.54,53.6 52.04,53.7 54.74,29 2.74,32.9 3.54,47.4 34.11,53.7 33.09,52.41 34.08,55.82 12.37,53.12 12.18,50.89 12.29,48.65 19.71,6.51 22.31,7.4 12.06,7.17 59.93,14.86 59.99,7.82 59.88,49.56 63.85,41.88 59.84,42.18 47.9,22.8 47.9,19.6 47.9,16.1 49.2,12.9 51.8,10.6 55,10.1 10.29,48.65 9.59,43.65 21.19,43.45 31.29,42.85 29.69,41.65 32.19,41.75 30.89,41.75 52.44,29 19.54,31.2 22.14,39.1 50.3,24.3 50.3,22.4 51.3,22.4 51.3,24.3 50.2,19.6 51.3,20.2 53.6,25.7 53.6,23.9 53.7,21.3 53.7,19.3 52,17.9 50.2,17.4 50.8,15.2 54.84,12.4 20.04,39.1 19.44,37 18.34,34.1 18.84,27.3 18.34,30 22.54,32 21.54,30.2 26.84,39.1 26.84,37.4 32.04,39.1 32.04,37.4 36.24,39.1 36.24,37.4 41.34,37.4 40.64,39.1 46.84,37.5 49.84,41.4 53.64,32.2 47.94,31.2 51.14,31 50.74,32.4 55.04,31 56.64,33 55.54,25.7 47.04,43.1 21.14,23.9 24.44,13.6 29.54,11.7 35.44,11.2 41.04,13.6 44.74,10.9 44.44,16.6 45.24,19.2 49.04,11.1 45.34,28.9 44.04,32.5 42.44,35.5 38.74,35.7 14.47,22.98 13.72,23.65 13.41,26.34 9.33,23.67 13.03,19.27 4.8,15.17 4.47,29.19 4.55,27.57 4.57,26.35 1.17,32.08 4.28,31.5 4.11,33.94 7.31,33.44 12.91,36.84 14.07,40.6 15.47,42.6 13.27,44.3 9.87,50.9 15.47,51 17.47,48.5 20.07,48.7 25.87,47.9 24.97,48.6 18.17,46.2 21.27,48.7 17.87,44.1 25.47,43.7 25.27,40.7 24.47,41.8 17.37,41.6 41.17,44.8 38.37,44.3 38.97,45.8 40.77,47.3 38.37,50.3 39.67,50.3 40.87,50.3 39.07,47.9 40.67,48.9 44.57,47.9 44.57,51.3 22.84,16 17.14,35.5 28.34,35.6 24.74,36.3 26.24,34.5
  pour Top (rank 2, no thermals): -0.8,1.9 -0.8,57.6 0.7,59.1 62.7,59.1 67.2,54.6 67.2,-0.4 65.4,-2.2 2.4,-2.2 -0.8,1
  pour Bottom (rank 2, no thermals): -1,1 -1,57.8 0.6,59.4 62.8,59.4 67.4,54.8 67.4,-0.7 65.7,-2.4 2.4,-2.4
  cutout Top: 48.6,28.4 48.6,19 49.7,19 49.7,28.4
  cutout Top: 51.9,28.4 53,28.4 53,20.3 51.9,20.3
  cutout Top: 44.4,39.1 45,39.7 45,40.9 46.7,42.6 47,42.3 45.6,40.9 45.6,40 45.6,39.5 44.8,38.7
GPS_1PPS  (via drill 0.3 pad 0.6)
  Top 0.2: U2.4 53.55,35.25 52.9,34.6 v46.9,34.6 | v40,42.91 39.85,42.75 33.44,42.75 31.73,44.46 26.74,44.46 25.33,45.87 25.33,47.17 24.53,47.97 R26.1 22.23,47.97 R31.1
  Bottom 0.2: v40,42.91 40.1,43.01 41.3,43.01 41.8,42.51 44.49,42.51 46.01,41 46.01,35.5 v46.9,34.6
GPS_RESET  (via drill 0.3 pad 0.6)
  Top 0.2: v18,10.19 18.3,10.49 18.3,14 16.82,15.47 R15.2
  Bottom 0.2: J6.P$22 31.17,1.15 29.82,2.5 29.82,3.32 29.12,4.01 28.27,4.01 27.4,4.88 27.4,7.6 25.7,9.29 19.41,9.29 19,9.7 18.51,10.19 v18,10.19 16.21,10.19 P9.P$1
GPS_RX  (via drill 0.3 pad 0.6)
  Top 0.2: U2.3 54.65,35.25 53.51,34.1 47.8,34.1 v47.6,33.9 47,33.9 46.39,33.29 46.39,32.32 46.7,32 46.7,11.9 46.3,11.5 R32.1 | D8.- 9.62,49.8 9.32,49.5 9.32,46.93 9.87,46.38 16.82,46.38 17.65,45.55 25.15,45.55 26.59,44.11 31.59,44.11 33.4,42.3 40.9,42.3 v41,42.4
  Bottom 0.2: v41,42.4 41.3,42.1 44.3,42.1 45.55,40.85 45.55,34.85 46.5,33.9 v47.6,33.9 48.6,34.9 P4.P$1
GPS_TX  (via drill 0.3 pad 0.6)
  Top 0.2: U2.2 55.75,35.45 53.95,33.65 48.45,33.65 47.8,33 v47.1,33 47.14,32.96 47.14,11.86 R29.1 | D9.- 9.87,52 8.77,50.9 8.77,46.78 9.53,46.02 16.68,46.02 17.5,45.2 25,45.2 26.44,43.76 31.44,43.76 33.55,41.65 40.25,41.65 v40.3,41.6
  Bottom 0.2: P5.P$1 48.7,32.7 48.4,33 v47.1,33 46.7,33 44.99,34.71 44.99,40.81 44.1,41.7 42.3,41.7 42.2,41.6 v40.3,41.6
GPS_WAKE_UP  (via drill 0.3 pad 0.6)
  Top 0.2: R19.1 18.7,14.45 18.7,9.79 v17,8.1
  Bottom 0.2: J6.P$32 17.2,2.1 17.2,7.89 v17,8.1 16.67,8.1 16.54,8.23 14.97,8.23 12.7,10.5 P11.P$1
I2C_SCL  (via drill 0.3 pad 0.6)
  Top 0.2: J3.30 14.87,25.6 15.29,26.02 v15.56,26.02 15.58,26 R11.1
  Bottom 0.2: J6.P$5 50.51,8.31 48.15,8.31 47,9.46 35.34,9.46 34.57,10.23 31.26,10.23 30.98,10.51 28.93,10.51 27.29,12.16 24.05,12.16 19.6,16.61 19.6,21.1 16.64,24.06 15.36,24.06 14.93,24.49 14.93,25.39 v15.56,26.02 17.26,26.02 P13.P$1
I2C_SDA  (via drill 0.3 pad 0.6)
  Top 0.2: R10.1 16.28,24.89 v15.56,24.89 15.47,24.8 J3.32
  Bottom 0.2: J6.P$3 53.03,7.33 51.7,8.66 48.39,8.66 47.15,9.9 35.4,9.9 34.71,10.58 31.4,10.58 31.12,10.87 29.08,10.87 27.43,12.51 24.2,12.51 19.95,16.76 19.95,21.25 19,22.2 P12.P$1 18.75,23.45 17.75,23.45 16.7,24.5 15.85,24.5 15.56,24.79 v15.56,24.89
LORA_3V3  (via drill 0.3 pad 0.6)
  Top 0.2: R34.2 14.57,47.57 v15.4,48.4
  Top 0.508: J3.24 13.92,28 14.64,27.28 17.55,27.28 18.09,26.74 R11.2 R10.2 | R37.2 14.39,54.23 R36.2 R35.2 | R9.2 25.94,46.78 25.94,46 26.97,44.97 31.94,44.97 33.65,43.26 39.06,43.26 39.5,43.7 v41,43.7 | U2.8 49.15,37.65 49.5,38 C8.2 48.5,38.7 | 48.5,38.7 C7.2 | v47.21,38.7 48.5,38.7
  Top 0.61: J3.39 4.83,22 5.73,22.9 5.73,22.09 4.84,21.2 J3.41 | 8.74,17.61 9.55,16.8 J3.52 | J3.24 8.12,28 8.1,28.02 v8.08,28.02 | 9.35,41.05 10.4,40 J3.2
  Top 1.016: 8.74,17.61 8.74,19.89 5.73,22.9 v5.73,28.02 5.73,37.43 9.35,41.05 11.5,43.2 14.6,43.2 v15.5,44.1 | R34.2 R35.2 25.7,49.8 27.09,48.41 R9.2
  Bottom 0.508: v41,43.7 41.5,43.7 42.19,43.01 44.7,43.01 46.61,41.11 46.61,39.3 v47.21,38.7
  Bottom 0.61: v8.08,28.02 v5.73,28.02
  Bottom 1.016: v15.5,44.1 15.3,44.3 15.3,47.5 v15.4,47.6 | v15.4,48.4 v16.3,48.4
  other vias: 14.6,44.3 14.9,43.5
  pour Top (no thermals): 14.7,47.2 15.8,47.2 16.7,48.1 16.7,49.1 16.4,49.4 15.7,50.1 15,50.1 14.5,50.1 14,49.6 14,47.5 14.3,47.2
  pour Bottom (no thermals): 14.8,47.3 14.8,48.6 15.1,48.9 16.6,48.9 16.7,48.8 16.9,48.6 16.9,48.1 16,47.2 15.8,47.2 14.9,47.2
  pour Top (no thermals): 13.9,43.7 13.9,44.4 14.1,44.6 15.7,44.6 15.9,44.4 16,44.3 16,43.9 14.8,42.7 14.2,42.7 13.9,43
  pour Bottom: 14.8,44.9 14.5,44.9 14.2,44.6 14.2,43.4 14.6,43 15.2,43 16,43.8 16,44.5 16,44.6 15.7,44.9
LR1302_RF
  Top 0.813: ANT2.D ANT3.SIG
N$1
  Top 0.2: J1.B5 50.73,48.62 50.9,48.44 R3.1
N$2
  Top 0.2: R4.2 53.72,47.24 J1.A5
N$3
  Top 0.508: U1.3 35.05,50.57 L1.1
  pour Top (no thermals): 34.76,51.56 34.76,49.25 35.2,48.81 37.35,48.81 37.63,49.09 37.63,49.78 37.18,50.23 36.01,50.23 35.5,50.74 35.5,51.48 35.31,51.67 34.87,51.67
N$4
  Top 0.406: R7.1 R8.2 32.71,53.2 U1.5
N$5
  Top 0.2: R6.1 R5.2 44.95,45.89 Q2.1
N$6  (via drill 0.3 pad 0.6)
  Top 0.508: v11.4,45.07 16.13,45.07 16.64,44.56 16.64,43.07 R12.1
  Bottom 0.508: J2.1 9.88,46.23 11.03,45.07 v11.4,45.07
N$11
  Top 0.2: U2.9 47.9,36.7 26.3,36.7 25.5,37.5 22.4,37.5 20.4,35.5 20.4,30.8 19.6,30 19.6,24.7 18.1,23.2 16.4,23.2 15.6,22.4 15.6,20.62 Q1.3
N$12
  Top 0.2: R15.1 R16.1 14.92,17.03 Q1.1
N$13
  Top 0.508: D6.- 16.57,40.44 R17.2
N$14
  Top 0.2: U2.5 52.45,35.55 51.9,35 47.7,35 46.35,36.35 26,36.35 25.25,37.1 22.5,37.1 20.75,35.35 20.75,30.65 19.95,29.85 19.95,24.55 18.2,22.8 17.3,22.8 16.57,22.07 R18.2
N$15
  Top 0.2: U2.18 arc45 56.74,27.08 R21.2
N$16
  Top 0.2: Q3.3 18.09,21.28 R18.1
N$17
  Top 0.2: R20.2 18.17,16.93 | 18.17,18.27 Q3.1 18.07,17.03 R20.2 | R19.2 R20.2
N$18
  Top 0.813: U2.11 C15.2 49.16,24.12 R24.1
N$19
  Top 0.813: R24.2 49.14,21.32 C9.2 49.13,20.05 C10.2
N$20
  Top 0.813: ANT1.SIG arc-45 62.74,11.4 63.3,11.4 arc-45 63.16,11.34 D5.2 54.48,11.34 arc-45 50.91,12.82 arc-45 49.14,17.1 C10.1 50.21,18.52 arc45 52,19.26 L2.2
N$21
  Top 0.813: U2.14 R22.1
N$22
  Top 0.813: R22.2 C11.2 52.45,21.25 L2.1
N$23  (via drill 0.3 pad 0.6)
  Top 0.2: R23.1 15.76,10.2 16.36,10.8 v16.7,10.8
  Bottom 0.2: J6.P$23 26.27,9.7 19.5,9.7 18.4,10.8 v16.7,10.8 15.9,11.6 15.9,13.5 P17.P$1
N$24  (via drill 0.3 pad 0.6)
  Top 0.2: R25.1 15.76,12.5 v17.1,12.5
  Bottom 0.2: J6.P$19 32.57,8.47 30.53,8.47 30.25,8.75 28.2,8.75 26.56,10.4 20.2,10.4 18.9,11.7 | 18.9,11.7 18.1,12.5 v17.1,12.5 | P15.P$1 18.9,11.7
N$25  (via drill 0.3 pad 0.6)
  Top 0.2: v17.5,11.5 17.4,11.6 15.56,11.6 R27.1
  Bottom 0.2: J6.P$21 30.1,8.4 28.06,8.4 26.41,10.05 19.85,10.05 18.6,11.3 17.7,11.3 v17.5,11.5 16.94,11.5 16.49,11.95 16.49,12.75 16.5,12.76 16.5,13.7 P16.P$1
N$27
  Top 0.2: R31.2 R33.2 20.67,46.31 Q5.1
N$28
  Top 0.2: R34.1 D7.+
N$29
  Top 0.2: D7.- 10.98,46.73 16.83,46.73 Q5.3
N$30
  Top 0.2: R35.1 D8.+
N$31
  Top 0.2: R37.1 D10.+
N$32
  Top 0.2: R36.1 D9.+
RPI_RX  (via drill 0.35)
  Top 0.2: v45.1,7.7 45.12,7.72 45.56,7.72 47.6,9.75 R29.2
  Bottom 0.2: J6.P$10 45.1,2.14 45.1,5.78 44.75,6.13 44.75,7.35 v45.1,7.7
RPI_TX  (via drill 0.35)
  Top 0.2: v45.5,8.65 46.3,9.45 R32.2
  Bottom 0.2: v45.5,8.65 47.15,8.65 47.7,8.1 47.7,2.08 J6.P$8
SPI_MISO
  Top 0.2: J3.47 1.75,18.8 1.15,18.2 1.15,12 2.45,10.7 13.14,10.7 R27.2
SPI_MOSI
  Top 0.2: J3.49 1.89,17.99 1.5,17.61 1.5,12.39 2.8,11.1 12.24,11.1 R25.2
SPI_SCK
  Top 0.2: J3.45 1.8,19.6 0.8,18.6 0.8,11.8 2.4,10.2 R23.2
SX1262_BUSY  (via drill 0.3 pad 0.6)
  Top 0.2: J3.8 13.5,37.6 v14.16,36.94
  Bottom 0.2: J6.P$12 42.56,2.14 42.56,3.54 42.03,4.07 40.91,4.07 40.1,4.88 40.1,7.61 39.13,8.58 35.22,8.58 34.3,9.5 34.27,9.53 30.97,9.53 30.68,9.81 28.64,9.81 27,11.46 23.76,11.46 18.9,16.32 18.9,20.8 16.35,23.35 15.05,23.35 14.14,24.26 14.14,36.92 v14.16,36.94 14.7,37.48 P6.P$1
SX1262_CSN  (via drill 0.3 pad 0.6)
  Top 0.2: v1.28,27.81 1.48,27.61 J3.25
  Bottom 0.2: J6.P$31 18.47,8.23 17.85,8.85 14.95,8.85 11.95,11.85 7.4,11.85 | 7.4,11.85 3.45,11.85 1.96,13.34 1.96,27.35 1.5,27.81 v1.28,27.81 | P19.P$1 7.4,11.85
SX1262_IO1  (via drill 0.3 pad 0.6)
  Top 0.2: J3.33 4.41,24.4 v4.5,24.31
  Bottom 0.2: J6.P$16 37.5,2.12 37.5,7.59 36.86,8.23 35.07,8.23 34.35,8.95 34.12,9.17 30.82,9.17 30.54,9.46 28.5,9.46 26.85,11.11 23.61,11.11 18.55,16.17 18.55,20.6 17.95,21.2 16,21.2 | 16,21.2 15.29,21.2 13.49,23 5.5,23 4.5,24 v4.5,24.31 | 16,21.2 15.9,21.3 P7.P$1
SX1262_IO2  (via drill 0.3 pad 0.6)
  Top 0.2: v4.5,25.2 J3.31
  Bottom 0.2: J6.P$18 34.9,2.18 34.9,7.9 33.98,8.82 30.67,8.82 30.39,9.11 28.35,9.11 26.7,10.75 23.36,10.75 18.11,16 18.11,20.39 17.8,20.7 15.18,20.7 | v4.5,25.2 4.21,25.2 3.87,24.86 3.87,24.07 5.34,22.6 13.28,22.6 15.18,20.7 | 15.18,20.7 15.18,19.98 P8.P$1
SX1262_RESET  (via drill 0.3 pad 0.6)
  Top 0.2: v6.8,30.58 6.51,30.87 6.51,35.38 7.93,36.8 J3.10
  Bottom 0.2: J6.P$29 20.01,7.33 18.14,9.2 15.1,9.2 12,12.3 7.5,12.3 | 7.5,12.3 3.6,12.3 2.36,13.54 2.36,28.52 4.42,30.58 v6.8,30.58 | P18.P$1 7.4,12.4 7.5,12.3
SX1302_CSN  (via drill 0.3 pad 0.6)
  Top 0.2: J3.51 3.96,17.2 5.6,15.56 5.6,12.3 6.4,11.5 11.7,11.5 v12.8,12.6
  Bottom 0.2: J6.P$24 27.28,2.18 27.28,3.32 26.5,4.1 25.2,4.1 24.8,4.5 24.8,7.8 23.76,8.84 19,8.84 18.29,9.55 15.25,9.55 12.8,12 v12.8,12.6 11.6,13.8 P10.P$1
SX1302_RESET  (via drill 0.3 pad 0.6)
  Top 0.2: v14.79,28.69 14.68,28.8 J3.22
  Bottom 0.2: J6.P$11 43.52,7.33 41.75,9.1 35.2,9.1 34.45,9.85 34.44,9.85 34.42,9.88 31.11,9.88 30.83,10.16 28.79,10.16 27.14,11.81 23.9,11.81 19.25,16.46 19.25,20.95 16.5,23.7 15.22,23.7 14.52,24.4 14.52,26.7 | v14.79,28.69 14.52,28.42 14.52,26.7 | 17.87,28.83 P14.P$1 16.2,26.7 14.52,26.7
USB_5V  (via drill 0.3 pad 0.6)
  Top 0.305: F2.2 46.06,47.6 R5.1
  Top 0.813: D1.+ 46,49.69 v46,51
  Top 1.016: F2.2 46,49.63 D1.+
  Bottom 0.813: P1.P$1 45.9,50.9 v46,51
V_BCKP  (via drill 0.3 pad 0.6)
  Top 0.508: v13.42,38.45 14.05,38.45 15.3,37.2 17.7,37.2 18.09,37.59 C13.2 | U2.6 51.35,37.65 50.8,38.2 C14.2 v51.8,38.7 | v46.05,42.75 44.7,41.4 44.7,39.8 44.01,39.11 42.89,39.11 42.06,39.94 19.64,39.94 19.2,39.5 19.2,38.7 18.8,38.3 C13.2 | R17.1 C13.2
  Bottom 0.508: v51.8,38.7 48.4,38.7 47.3,39.8 47.3,41.49 v46.05,42.75
  Bottom 0.61: v13.42,38.45 10.46,38.45 J8.P$1

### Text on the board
tPlace: LR1302 LoRaWAN HAT for RPI V1.0 | GND | IO26 | IO19 | IO13 | IO6 | IO5 | SDA0 | GND | SCK | MISO | MOSI | 3V3 | IO22 | IO27 | IO17 | GND | IO4 | SCL | SDA | 3V3 | RX | TX | 5V | 5V | IO21 | IO20 | IO16 | GND | IO12 | GND | SCL0 | CE1 | CE0 | IO25 | GND | IO24 | IO23 | GND | IO18 | GND
bNames: J6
